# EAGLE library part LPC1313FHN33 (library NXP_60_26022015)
32-bit ARM Cortex-M3 microcontroller; up to 32 kB flash and 8 kB SRAM; USB device The LPC1311/13/42/43 are ARM Cortex-M3 based microcontrollers for embedded applications featuring a high level of integration and low power consumption. The ARM Cortex-M3 is a next generation core that offers system enhancements such as enhanced debug features and a higher level of support block integration. The LPC1311/13/42/43 operate at CPU frequencies of up to 72 MHz. The ARM Cortex-M3 CPU incorporates a 3-stage pipeline and uses a Harvard architecture with separate local instruction and data buses as well as a third bus for peripherals. The ARM Cortex-M3 CPU also includes an internal prefetch unit that supports speculative branching. The peripheral complement of the LPC1311/13/42/43 includes up to 32 kB of flash memory, up to 8 kB of data memory, USB Device (LPC1342/43 only), one Fast-mode Plus I 2 C-bus interface, one UART, four general purpose timers, and up to 42 general purpose I/O pins. Remark: The LPC1311/13/42/43 series consists of the LPC1300 series (parts LPC1311/13/42/43) and the LPC1300L series (parts LPC1311/01 and LPC1313/01). The LPC1300L series features the following enhancements over the LPC1300 series: Power profiles with lower power consumption in Active and Sleep modes. Four levels for BOD forced reset. Second SSP controller (LPC1313FBD48/01 only). Windowed Watchdog Timer (WWDT). Internal pull-up resistors pull up pins to full VDD level. Programmable pseudo open-drain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
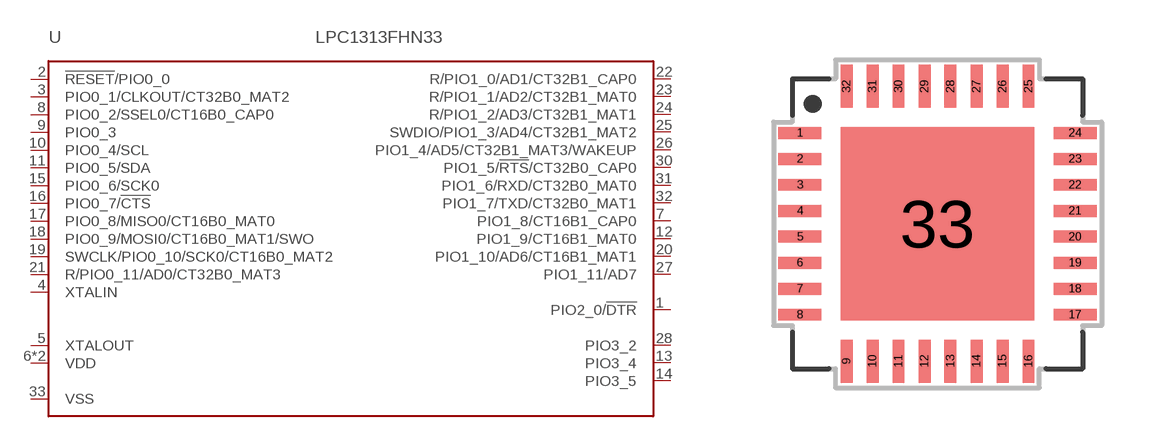
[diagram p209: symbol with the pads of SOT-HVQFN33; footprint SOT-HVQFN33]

Designator prefix U

## LPC1313FHN33 (ADC: 8; FLASH: 32kB; PWR_PROFILES: no; SERIES: LPC1300; SRAM: 8kB; SSP: 1; USB: -), LPC1313FHN33/01 (ADC: 8; FLASH: 32kB; PWR_PROFILES: yes; SERIES: LPC1300L; SRAM: 8kB; SSP: 1; USB: -)  [SOT-HVQFN33]
1  PIO2_0/!DTR!
2  !RESET!/PIO0_0
3  PIO0_1/CLKOUT/CT32B0_MAT2
4  XTALIN  in
5  XTALOUT  out
6  VDD  pwr
7  PIO1_8/CT16B1_CAP0
8  PIO0_2/SSEL0/CT16B0_CAP0
9  PIO0_3
10  PIO0_4/SCL
11  PIO0_5/SDA
12  PIO1_9/CT16B1_MAT0
13  PIO3_4
14  PIO3_5
15  PIO0_6/SCK0
16  PIO0_7/!CTS!
17  PIO0_8/MISO0/CT16B0_MAT0
18  PIO0_9/MOSI0/CT16B0_MAT1/SWO
19  SWCLK/PIO0_10/SCK0/CT16B0_MAT2
20  PIO1_10/AD6/CT16B1_MAT1
21  R/PIO0_11/AD0/CT32B0_MAT3
22  R/PIO1_0/AD1/CT32B1_CAP0
23  R/PIO1_1/AD2/CT32B1_MAT0
24  R/PIO1_2/AD3/CT32B1_MAT1
25  SWDIO/PIO1_3/AD4/CT32B1_MAT2
26  PIO1_4/AD5/CT32B1_MAT3/WAKEUP
27  PIO1_11/AD7
28  PIO3_2
29  VDD  pwr
30  PIO1_5/!RTS!/CT32B0_CAP0
31  PIO1_6/RXD/CT32B0_MAT0
32  PIO1_7/TXD/CT32B0_MAT1
33  VSS  pwr

## Footprint SOT-HVQFN33 (pad centres in mm)
SOTxxx HVQFN33: plastic thermal enhanced very thin quad flat package; no leads; 33 terminals; body 7 x 7 x 0.85 mm JEDEC: --- IEC: --- Package according LPC111x datasheet
smd 1.075 x 0.3: 1 -3.438,2.275; 2 -3.438,1.625; 3 -3.438,0.975; 4 -3.438,0.325; 5 -3.438,-0.325; 6 -3.438,-0.975; 7 -3.438,-1.625; 8 -3.438,-2.275; 17 3.438,-2.275; 18 3.438,-1.625; 19 3.438,-0.975; 20 3.438,-0.325; 21 3.438,0.325; 22 3.438,0.975; 23 3.438,1.625; 24 3.438,2.275
smd 0.3 x 1.075: 9 -2.275,-3.438; 10 -1.625,-3.438; 11 -0.975,-3.438; 12 -0.325,-3.438; 13 0.325,-3.438; 14 0.975,-3.438; 15 1.625,-3.438; 16 2.275,-3.438; 25 2.275,3.438; 26 1.625,3.438; 27 0.975,3.438; 28 0.325,3.438; 29 -0.325,3.438; 30 -0.975,3.438; 31 -1.625,3.438; 32 -2.275,3.438
smd 4.85 x 4.85: 33 0,0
